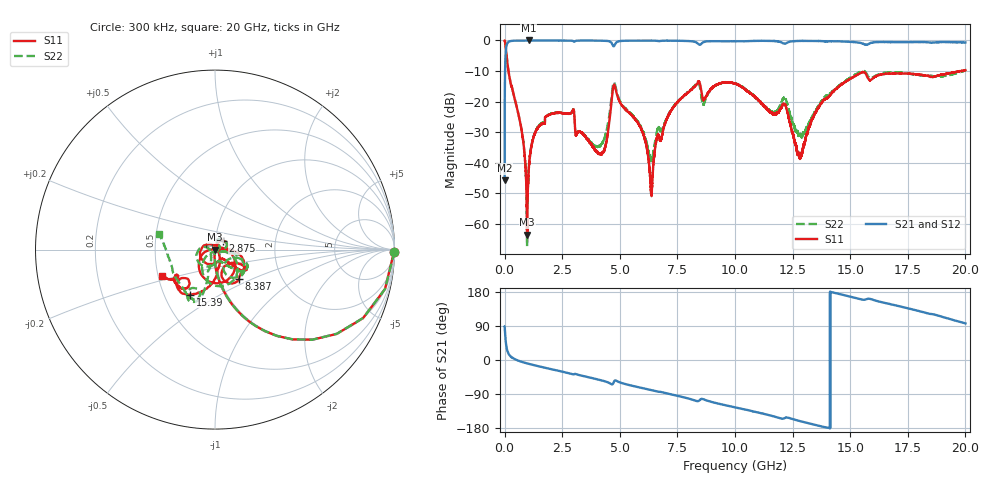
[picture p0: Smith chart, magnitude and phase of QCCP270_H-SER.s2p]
!{QCCP270}
!Johanson Technology Inc.
!www.johansontechnology.com
!Test Board Conditions:
!Substrate Type  RO4350B
!Substrate Thickness  20 mil
!Substrate Dk  3.66
!TL Type: GCPW
!TL Trace Width  36 mil
!TL Gap  12 mil
!Electrode orientation  Horizontal
!DUT TOPOLOGY	SERIES
!Mounting Pad LxW  26x36 mil
! Created Sat Jan  9 18:34:50 2021
# hz S ma R 50
! 2 Port Network Data from SP1.SP block
! freq  magS11  angS11  magS21  angS21  magS12  angS12  magS22  angS22
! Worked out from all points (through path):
!   20001 points, 300 kHz to 20 GHz, reference 50 ohm
!   highest |S21| = 0.00 dB at 1.053 GHz (marker M1); lowest = -45.6 dB at 300 kHz (marker M2)
!   group delay of S21, straight-line fit = 36.5 ps
!   lowest |S11| = -63.5 dB at 975.3 MHz (marker M3), VSWR 1.00, Z = 50.1 - j0.024 ohm
!   |S11| at or under -10 dB: 167.9 MHz to 19.81 GHz (19.64 GHz wide, 197 % of centre); 19.81712 GHz to 19.81924 GHz (2.119 MHz wide, 0.0107 % of centre)
!   |S22| runs from -67.2 to 0.0 dB; largest |S21 - S12| = 0.016
!   S11 on the Smith chart (normalised r, x): 300 kHz: open; 2.875 GHz: 1.08, +0.11; 8.387 GHz: 1.23, -0.42; 15.39 GHz: 0.68, -0.37; 20 GHz: 0.53, -0.17
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300000  0.9978 -0.6  0.005221 88.5  0.005292 88.8  1 -0.6
1.363e8  0.3832 -68.6  0.9213 21.3  0.9219 21.2  0.3839 -68.4
7.343e8  0.03493 -93.9  0.9974 -4.6  0.9969 -4.6  0.03485 -93.9
9.753e8  0.0006704 -21.0  0.9985 -8.9  0.9983 -8.9  0.0004349 -30.6
1.0533e9  0.008473 75.6  0.9996 -10.2  0.9979 -10.2  0.008492 79.6
1.4503e9  0.03755 71.0  0.9969 -16.2  0.9969 -16.2  0.03867 74.6
2.8753e9  0.06479 48.5  0.9918 -36.1  0.9917 -36.1  0.06503 53.5
3.3343e9  0.03129 51.6  0.995 -41.2  0.9949 -41.2  0.03148 40.1
4.2583e9  0.01453 65.2  0.9911 -54.6  0.9905 -54.6  0.02142 -19.2
4.7753e9  0.1833 -97.4  0.8391 -54.5  0.8401 -54.5  0.2006 -90.3
5.9603e9  0.03332 -175.3  0.9944 -73.9  0.9944 -73.9  0.03509 -142.7
6.3513e9  0.003749 111.9  0.9943 -79.3  0.9936 -79.3  0.01112 -81.8
6.6673e9  0.02846 -19.5  0.9795 -83.6  0.9784 -83.6  0.03777 -33.3
8.3873e9  0.2121 -50.8  0.8915 -108.6  0.8898 -108.5  0.1961 -40.0
8.6483e9  0.1067 -53.2  0.9442 -104.0  0.9442 -104.0  0.09103 -36.7
1.00003e10  0.1975 -35.7  0.9716 -125.1  0.9707 -125.2  0.1978 -35.8
1.21553e10  0.0908 -150.3  0.8849 -153.3  0.886 -153.3  0.1153 -147.2
1.28003e10  0.01283 37.8  0.9823 -160.8  0.9837 -160.9  0.02881 -171.6
1.33343e10  0.05035 -58.7  0.9824 -169.0  0.9844 -169.0  0.05549 -113.4
1.53903e10  0.2858 -118.6  0.9204 161.2  0.9253 160.9  0.3001 -108.5
1.66673e10  0.2859 -132.8  0.9413 148.3  0.9316 148.2  0.3007 -112.5
2e10  0.3278 -153.6  0.9277 96.6  0.9178 96.4  0.3264 164.0
